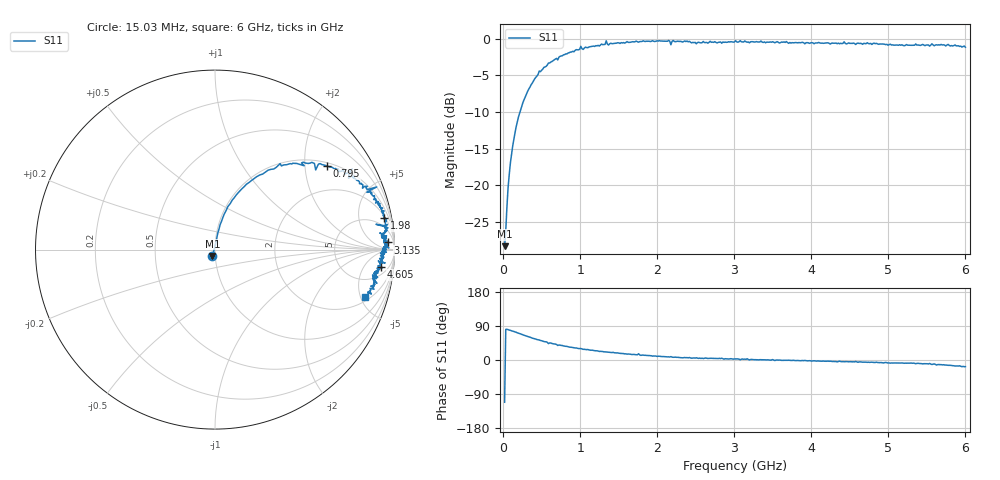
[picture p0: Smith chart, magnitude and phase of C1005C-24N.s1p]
!	Network	Analyzer	HP8753E.07.74:	Oct	30	2002	Serial	No.	JP38451487
!	Hewlett-Packard
!	7	Sep	2009	9:00:17
!	Frequency	S11
#	HZ	S	RI	R	50
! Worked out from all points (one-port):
!   400 points, 15.03 MHz to 6 GHz, reference 50 ohm
!   lowest |S11| = -28.3 dB at 15.03 MHz (marker M1), VSWR 1.08, Z = 48.5 - j3.48 ohm
!   |S11| at or under -10 dB: start of sweep to 215.8 MHz
!   S11 on the Smith chart (normalised r, x): 15.03 MHz: 0.97, -0.07; 795 MHz: 1.11, +2.61; 1.98 GHz: 2, +10; 3.135 GHz: 24, +27; 4.605 GHz: 9, -13; 6 GHz: 2.44, -5.42
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1.502992e7  -0.0141 -0.0358
3.002985e7  0.00782 0.0484
6.00297e7  0.0164 0.0948
9.002955e7  0.0286 0.139
1.95029e8  0.0962 0.276
4.650277e8  0.363 0.479
7.650262e8  0.6 0.473
7.95026e8  0.625 0.464
1.005025e9  0.764 0.447
1.320023e9  0.85 0.335
1.335023e9  0.901 0.349
1.365023e9  0.846 0.319
1.515022e9  0.884 0.279
1.740021e9  0.925 0.227
1.755021e9  0.906 0.269
1.785021e9  0.934 0.202
1.98002e9  0.943 0.174
2.145019e9  0.961 0.14
2.175019e9  0.897 0.141
2.205019e9  0.964 0.121
2.265019e9  0.953 0.118
3.015015e9  0.966 0.0462
3.135014e9  0.963 0.0398
3.765011e9  0.936 -0.0125
4.515007e9  0.926 -0.072
4.605007e9  0.927 -0.0972
5.265004e9  0.892 -0.13
6e9  0.833 -0.263
